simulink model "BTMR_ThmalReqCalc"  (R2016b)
settings: Solver=FixedStepDiscrete  StartTime=0.0  StopTime=10.0  FixedStep=0.1  RelTol=1e-3  EnableMultiTasking=on
undefined symbols (not defined in the file or in its folder): BMS_cntThmStbNum_C, BTMR_cntThmalReqVal_C, BTMR_flgCoolPwrCal_C, BTMR_pChrgClntPwrLv1_C, BTMR_pChrgClntPwrLv2_C, BTMR_pChrgClntPwrLv3_C, BTMR_pChrgClntPwrLv4_C, BTMR_pChrgClntPwrLv5_C, BTMR_pChrgClntPwrLv6_C, BTMR_pCoolPwrVal_C, BTMR_pHtgACPwrReq_C, BTMR_pHtgDCPwrReq_C, BTMR_pHtgDrvPwrReq_C, BTMR_pHtgsStage1_CUR, BTMR_pHtgsStage2_CUR, BTMR_pNormClntPwrLv1_C, BTMR_pNormClntPwrLv2_C, BTMR_pNormClntPwrLv3_C, BTMR_r861BrsDrvSoc_C, BTMR_r861HtgDrvSoc_C, BTMR_r891BrsDrvSoc_C, BTMR_r891HtgDrvSoc_C, BTMR_rCoolClbFlg_C, BTMR_rFlashClbFlg_C, BTMR_rHeatClbFlg_C, BTMR_t861BrsDiffLv0Temp_C, BTMR_t861BrsDiffLv1Temp_C, BTMR_t861CoolChrgAces2Temp_C, BTMR_t861CoolChrgAces3Temp_C, BTMR_t861CoolChrgAcesTemp_C, BTMR_t861CoolChrgDiffDebTemp_C, BTMR_t861CoolChrgEndDiffTemp_C, BTMR_t861CoolChrgExitLv2Temp_C, BTMR_t861CoolChrgExitLv3Temp_C, BTMR_t861CoolChrgExitTemp_C, BTMR_t861CoolChrgIntLv0Temp_C, BTMR_t861CoolChrgIntLv1Temp_C, BTMR_t861CoolChrgIntLv2Temp_C, BTMR_t861CoolChrgIntLv3Temp_C, BTMR_t861CoolChrgIntLv4Temp_C, BTMR_t861CoolChrgIntLv5Temp_C, BTMR_t861CoolDCDebTemp_C, BTMR_t861CoolNormAcesTemp_C, BTMR_t861CoolNormDiffDebTemp_C, BTMR_t861CoolNormEndDiffTemp_C, BTMR_t861CoolNormExitLv2Temp_C, BTMR_t861CoolNormExitLv3Temp_C, BTMR_t861CoolNormExitTemp_C, BTMR_t861CoolNormIntLv0Temp_C, BTMR_t861CoolNormIntLv1Temp_C, BTMR_t861CoolNormLv2Temp_C, BTMR_t861CoolNormLv3Temp_C, BTMR_t861HtgACDiffDebTemp_C, BTMR_t861HtgACEndDiffTemp_C, BTMR_t861HtgACStartHiTemp_C, BTMR_t861HtgACStartLoTemp_C, BTMR_t861HtgACStopTemp_C, BTMR_t861HtgDCDiffDebTemp_C, BTMR_t861HtgDCEndDiffTemp_C, BTMR_t861HtgDCIntLv0Temp_C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
libraries: AIWAYS_Powertrain_BMS_lib x78, simulink x9
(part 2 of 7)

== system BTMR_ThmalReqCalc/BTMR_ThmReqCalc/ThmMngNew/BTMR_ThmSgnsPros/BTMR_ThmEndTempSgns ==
  BSPR_tCellTempMin : Inport
  BSPR_tCellTempMax : Inport  Port=2
  BCMR_bAcChrgHeatFbd : Inport  Port=3
  DSMR_stFaultRank : Inport  Port=4
  BMCR_stBmsModeCtrl : Inport  Port=5
  COMR_bLeadAcidChgHvOn : Inport  Port=6
  BTMR_flgBMSSgns : Inport  Port=7
  BTMR_CoolChrgThmEndCalc : Subsystem
  BTMR_CoolNormThmEndCalc : Subsystem
  BTMR_HtgACThmEndCalc : Subsystem
  BTMR_HtgDCThmEndCalc : Subsystem
  BTMR_HtgDrvThmEndCalc : Subsystem
  BTMR_ThmEndComCalc : Subsystem
  Bus Creator : BusCreator  Inputs=6
  Logical Operator{1..4,10} (5 alike) : Logic  Operator=OR  AllPortsSameDT=off  OutDataTypeStr=boolean
  BTMR_flgThmEndSgns : Outport
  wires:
  BMCR_stBmsModeCtrl/1 -> BTMR_ThmEndComCalc/1(BMCR_stBmsModeCtrl)
  DSMR_stFaultRank/1 -> BTMR_ThmEndComCalc/2(DSMR_stFaultRank)
  BTMR_ThmEndComCalc/1(BTMR_ThmEndCom) -> Logical Operator10/1, Logical Operator4/1, Logical Operator3/1, Logical Operator2/1, Logical Operator1/1, Bus Creator/1  "BTMR_flgBrsThmEnd"
  BTMR_flgBMSSgns/1 -> BTMR_CoolChrgThmEndCalc/1(BTMR_flgBMSSgns), BTMR_CoolNormThmEndCalc/1(BTMR_flgBMSSgns), BTMR_HtgDrvThmEndCalc/1(BTMR_flgBMSSgns), BTMR_HtgACThmEndCalc/1(BTMR_flgBMSSgns), BTMR_HtgDCThmEndCalc/1(BTMR_flgBMSSgns)
  BSPR_tCellTempMax/1 -> BTMR_CoolChrgThmEndCalc/2(BSPR_tCellTempMax), BTMR_CoolNormThmEndCalc/2(BSPR_tCellTempMax), BTMR_HtgDrvThmEndCalc/2(BSPR_tCellTempMax), BTMR_HtgACThmEndCalc/2(BSPR_tCellTempMax), BTMR_HtgDCThmEndCalc/2(BSPR_tCellTempMax)
  BSPR_tCellTempMin/1 -> BTMR_CoolChrgThmEndCalc/3(BSPR_tCellTempMin), BTMR_CoolNormThmEndCalc/3(BSPR_tCellTempMin), BTMR_HtgDrvThmEndCalc/3(BSPR_tCellTempMin), BTMR_HtgACThmEndCalc/3(BSPR_tCellTempMin), BTMR_HtgDCThmEndCalc/3(BSPR_tCellTempMin)
  BTMR_HtgDCThmEndCalc/1(BTMR_HtgDCThmEnd) -> Logical Operator10/2
  BTMR_HtgACThmEndCalc/1(BTMR_HtgACThmEnd) -> Logical Operator1/2
  BTMR_HtgDrvThmEndCalc/1(BTMR_HtgDrvThmEnd) -> Logical Operator2/2
  BTMR_CoolNormThmEndCalc/1(BTMR_CoolNormThmEnd) -> Logical Operator3/2
  BTMR_CoolChrgThmEndCalc/1(BTMR_CoolChrgThmEnd) -> Logical Operator4/2
  Logical Operator10/1 -> Bus Creator/2  "BTMR_flgHtgDCThmEnd"
  Logical Operator1/1 -> Bus Creator/3  "BTMR_flgHtgACThmEnd"
  Logical Operator2/1 -> Bus Creator/4  "BTMR_flgHtgDrvThmEnd"
  Logical Operator3/1 -> Bus Creator/5  "BTMR_flgCoolNormThmEnd"
  Logical Operator4/1 -> Bus Creator/6  "BTMR_flgCoolChrgThmEnd"
  Bus Creator/1 -> BTMR_flgThmEndSgns/1  "BTMR_flgThmEndSgns"
  COMR_bLeadAcidChgHvOn/1 -> BTMR_ThmEndComCalc/3(COMR_bLeadAcidChgHvOn)
  BCMR_bAcChrgHeatFbd/1 -> BTMR_HtgACThmEndCalc/4(BCMR_bAcChrgHeatFbd)

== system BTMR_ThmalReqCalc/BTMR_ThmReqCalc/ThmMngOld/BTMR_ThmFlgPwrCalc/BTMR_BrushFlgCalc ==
  stBrsSts : Inport
  Constant1 : Constant  Value=enmThmBrsFlg.INACTIVE  OutDataTypeStr=Enum: enmThmBrsFlg
  Constant2 : Constant  Value=BTMR_cntThmalReqVal_C
  Constant21 : Constant  Value=enmThmBrsSts.ACTIVE  OutDataTypeStr=Enum: enmThmBrsSts
  Constant3 : Constant  Value=enmThmBrsFlg.ACTIVE  OutDataTypeStr=Enum: enmThmBrsFlg
  Data Type Conversion : DataTypeConversion  OutDataTypeStr=uint8
  Data Type Conversion1 : DataTypeConversion  OutDataTypeStr=uint8
  Data Type Conversion2 : DataTypeConversion  OutDataTypeStr=uint8
  Relational Operator7 : RelationalOperator  Operator===  OutDataTypeStr=boolean  RndMeth=Simplest
  Stable_Calc1 : Subsystem
  Switch1 : Switch  Criteria=u2 ~= 0
  BTMR_flgBrsPwrReq : Outport
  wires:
  Data Type Conversion2/1 -> Switch1/3
  stBrsSts/1 -> Relational Operator7/1
  Data Type Conversion1/1 -> Switch1/1
  Relational Operator7/1 -> Stable_Calc1/1(source_Uint)
  Constant21/1 -> Data Type Conversion/1
  Switch1/1 -> BTMR_flgBrsPwrReq/1
  Data Type Conversion/1 -> Relational Operator7/2
  Constant3/1 -> Data Type Conversion1/1
  Constant1/1 -> Data Type Conversion2/1
  Constant2/1 -> Stable_Calc1/2(cntStable)
  Stable_Calc1/1(stableOut) -> Switch1/2

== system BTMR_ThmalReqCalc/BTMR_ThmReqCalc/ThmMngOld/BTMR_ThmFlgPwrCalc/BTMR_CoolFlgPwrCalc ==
  BTMR_flgBrsPwrReq : Inport
  stCoolSts : Inport  Port=2
  BTMR_flgCoolTempSgns : Inport  Port=3
  BTMR_CoolChrgFlgPwrCalc : Subsystem
  BTMR_CoolNormFlgPwrCalc : Subsystem
  BTMR_flgPow_Out : Subsystem
  Bus Selector1 : BusSelector  OutputSignals=BTMR_flgCoolNormTempSgns,BTMR_flgCoolChrgTempSgns
  Constant1 : Constant  Value=enmThmCoolSts.CoolChrg  OutDataTypeStr=Enum: enmThmCoolSts
  Constant13 : Constant  Value=enmThmCoolSts.CoolNorm  OutDataTypeStr=Enum: enmThmCoolSts
  Data Type Conversion : DataTypeConversion  OutDataTypeStr=uint8
  Data Type Conversion1 : DataTypeConversion  OutDataTypeStr=uint8
  Merge : Merge
  Merge1 : Merge
  Relational Operator2 : RelationalOperator  Operator===  OutDataTypeStr=boolean  RndMeth=Simplest
  Relational Operator3 : RelationalOperator  Operator===  OutDataTypeStr=boolean  RndMeth=Simplest
  BTMR_flgClntPwrReq : Outport
  BTMR_pClntPwrReq : Outport  Port=2
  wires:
  Relational Operator3/1 -> BTMR_CoolChrgFlgPwrCalc/Enable
  stCoolSts/1 -> [stCoolSts], Relational Operator2/1, Relational Operator3/1
  Data Type Conversion1/1 -> Relational Operator3/2
  Relational Operator2/1 -> BTMR_CoolNormFlgPwrCalc/Enable
  Constant13/1 -> Data Type Conversion/1
  BTMR_flgCoolTempSgns/1 -> Bus Selector1/1
  BTMR_flgPow_Out/1(BTMR_flgClntPwrReq) -> BTMR_flgClntPwrReq/1
  BTMR_flgPow_Out/2(BTMR_pClntPwrReq) -> BTMR_pClntPwrReq/1
  Bus Selector1/1 -> BTMR_CoolNormFlgPwrCalc/1(BTMR_flgCoolNormTempSgns)  "<BTMR_flgCoolNormTempSgns>"
  Bus Selector1/2 -> BTMR_CoolChrgFlgPwrCalc/1(BTMR_flgCoolChrgTempSgns)  "<BTMR_flgCoolChrgTempSgns>"
  BTMR_flgBrsPwrReq/1 -> BTMR_flgPow_Out/2(BTMR_flgBrsPwrReq)
  Data Type Conversion/1 -> Relational Operator2/2
  Constant1/1 -> Data Type Conversion1/1
  BTMR_CoolNormFlgPwrCalc/1(BTMR_flgClntPwrReq) -> Merge/1
  BTMR_CoolChrgFlgPwrCalc/1(BTMR_flgClntPwrReq) -> Merge/2
  BTMR_CoolNormFlgPwrCalc/2(BTMR_pClntPwrReq) -> Merge1/1
  Merge/1 -> BTMR_flgPow_Out/3(BTMR_flgClntPwrReqMerge)
  BTMR_CoolChrgFlgPwrCalc/2(BTMR_pClntPwrReq) -> Merge1/2
  [stCoolSts] -> BTMR_flgPow_Out/1(stCoolSts)
  Merge1/1 -> BTMR_flgPow_Out/4(BTMR_pClntPwrReqMerge)

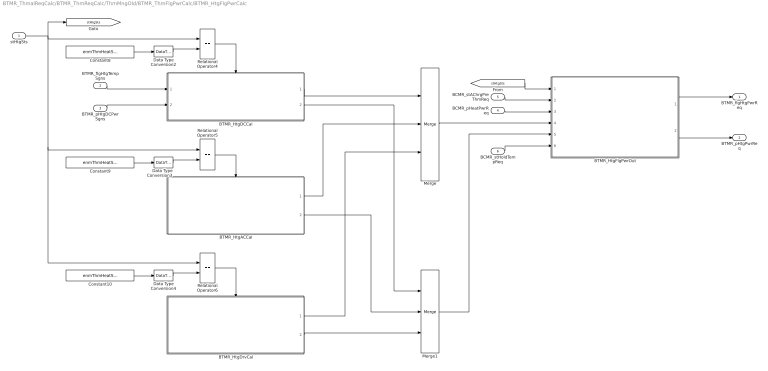
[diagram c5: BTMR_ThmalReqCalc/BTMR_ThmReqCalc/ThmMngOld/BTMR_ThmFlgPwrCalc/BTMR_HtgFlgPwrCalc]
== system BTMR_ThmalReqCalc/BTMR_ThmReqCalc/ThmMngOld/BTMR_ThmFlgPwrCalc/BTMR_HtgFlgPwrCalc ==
  stHtgSts : Inport
  BTMR_flgHtgTempSgns : Inport  Port=2
  BTMR_pHtgDCPwrSgns : Inport  Port=3
  BCMR_pHeatPwrReq : Inport  Port=4
  BCMR_stAChrgPreThmReq : Inport  Port=5
  BCMR_stHoldTempReq : Inport  Port=6
  BTMR_HtgACCal : Subsystem
  BTMR_HtgDCCal : Subsystem
  BTMR_HtgDrvCal : Subsystem
  BTMR_HtgFlgPwrOut : Subsystem
  Constant10 : Constant  Value=enmThmHeatSts.HeatDrv  OutDataTypeStr=Enum: enmThmHeatSts
  Constant8 : Constant  Value=enmThmHeatSts.HeatDC  OutDataTypeStr=Enum: enmThmHeatSts
  Constant9 : Constant  Value=enmThmHeatSts.HeatAC  OutDataTypeStr=Enum: enmThmHeatSts
  Data Type Conversion2 : DataTypeConversion  OutDataTypeStr=uint8
  Data Type Conversion3 : DataTypeConversion  OutDataTypeStr=uint8
  Data Type Conversion4 : DataTypeConversion  OutDataTypeStr=uint8
  Merge : Merge  Inputs=3
  Merge1 : Merge  Inputs=3
  Relational Operator4 : RelationalOperator  Operator===  OutDataTypeStr=boolean  RndMeth=Simplest
  Relational Operator5 : RelationalOperator  Operator===  OutDataTypeStr=boolean  RndMeth=Simplest
  Relational Operator6 : RelationalOperator  Operator===  OutDataTypeStr=boolean  RndMeth=Simplest
  BTMR_flgHtgPwrReq : Outport
  BTMR_pHtgPwrReq : Outport  Port=2
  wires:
  stHtgSts/1 -> [stHtgSts], Relational Operator6/1, Relational Operator5/1, Relational Operator4/1
  Relational Operator6/1 -> BTMR_HtgDrvCal/Enable
  BTMR_flgHtgTempSgns/1 -> BTMR_HtgDCCal/1(BTMR_flgHtgDCCalSgns)
  BTMR_pHtgDCPwrSgns/1 -> BTMR_HtgDCCal/2(BTMR_pHtgDCPowCur)
  Relational Operator4/1 -> BTMR_HtgDCCal/Enable
  Data Type Conversion2/1 -> Relational Operator4/2
  Constant8/1 -> Data Type Conversion2/1
  Data Type Conversion3/1 -> Relational Operator5/2
  Constant9/1 -> Data Type Conversion3/1
  Data Type Conversion4/1 -> Relational Operator6/2
  Constant10/1 -> Data Type Conversion4/1
  Relational Operator5/1 -> BTMR_HtgACCal/Enable
  BTMR_HtgDCCal/1(BTMR_flgHtgPwrReq) -> Merge/1
  BTMR_HtgACCal/1(BTMR_flgHtgPwrReq) -> Merge/2
  BTMR_HtgDrvCal/1(BTMR_flgHtgPwrReq) -> Merge/3
  BTMR_HtgDrvCal/2(BTMR_pHtgPwrReq) -> Merge1/3
  BTMR_HtgDCCal/2(BTMR_pHtgPwrReq) -> Merge1/1
  BTMR_HtgACCal/2(BTMR_pHtgPwrReq) -> Merge1/2
  BCMR_stAChrgPreThmReq/1 -> BTMR_HtgFlgPwrOut/2(BCMR_stAChrgPreThmReq)
  Merge/1 -> BTMR_HtgFlgPwrOut/4(BTMR_flgHtgPwrReqMerge)
  [stHtgSts] -> BTMR_HtgFlgPwrOut/1(stHtgSts)
  BCMR_pHeatPwrReq/1 -> BTMR_HtgFlgPwrOut/3(BCMR_pHeatPwrReq)
  Merge1/1 -> BTMR_HtgFlgPwrOut/5(BTMR_pHtgPwrReqMerge)
  BTMR_HtgFlgPwrOut/1(BTMR_flgHtgPwrReq) -> BTMR_flgHtgPwrReq/1
  BTMR_HtgFlgPwrOut/2(BTMR_pHtgPwrReq) -> BTMR_pHtgPwrReq/1
  BCMR_stHoldTempReq/1 -> BTMR_HtgFlgPwrOut/6(BCMR_stHoldTempReq)

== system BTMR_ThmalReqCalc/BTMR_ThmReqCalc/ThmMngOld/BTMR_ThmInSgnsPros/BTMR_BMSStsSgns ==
  COMR_bLeadAcidChgHvOn : Inport
  BMCR_stBmsModeCtrl : Inport  Port=2
  BSER_rSoc : Inport  Port=3
  BTMR_BmsStsCalc : Subsystem
  BTMR_SOCStsCalc : Subsystem
  BTMR_flgBMSSgns : Outport
  BTMR_flgSOCSgns : Outport  Port=2
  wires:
  BSER_rSoc/1 -> BTMR_SOCStsCalc/1(BSER_rSoc)
  BMCR_stBmsModeCtrl/1 -> BTMR_BmsStsCalc/1(BMCR_stBmsModeCtrl)
  BTMR_SOCStsCalc/1(BTMR_flgSOCSgns) -> BTMR_flgSOCSgns/1
  BTMR_BmsStsCalc/1(BTMR_flgBMSSgns) -> BTMR_flgBMSSgns/1
  COMR_bLeadAcidChgHvOn/1 -> BTMR_BmsStsCalc/2(COMR_bLeadAcidChgHvOn)

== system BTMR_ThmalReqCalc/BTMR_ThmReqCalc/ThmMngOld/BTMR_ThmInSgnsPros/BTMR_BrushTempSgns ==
  BSPR_tCellTempMin : Inport
  BSPR_tCellTempMax : Inport  Port=2
  BSPR_tClntUsT : Inport  Port=3
  BTMR_BrsDnaTempCalc : Subsystem
  BTMR_BrsEna1TempCalc : Subsystem
  BTMR_BrsEna2TempCalc : Subsystem
  BTMR_BrsEna3TempCalc : Subsystem
  BTMR_BrsIntEna1TempCalc : Subsystem
  BTMR_BrsIntEna2TempCalc : Subsystem
  BTMR_BrsIntEna3TempCalc : Subsystem
  BTMR_BrsStartTempCalc : Subsystem
  Bus Creator : BusCreator  Inputs=2
  Bus Creator1 : BusCreator  Inputs=3
  Bus Creator2 : BusCreator  Inputs=3
  Bus Creator3 : BusCreator  Inputs=3
  BTMR_flgBrsTempSgns : Outport
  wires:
  BTMR_BrsEna2TempCalc/1(BTMR_flgBrsEna2Temp) -> Bus Creator1/2  "BTMR_flgBrsEna2Temp"
  BTMR_BrsEna1TempCalc/1(BTMR_flgBrsEna1Temp) -> Bus Creator1/1  "BTMR_flgBrsEna1Temp"
  BTMR_BrsStartTempCalc/1(BTMR_flgBrsStartTemp) -> Bus Creator/1  "BTMR_flgBrsStartTemp"
  BSPR_tCellTempMin/1 -> BTMR_BrsEna3TempCalc/1(BSPR_tCellTempMin), BTMR_BrsEna2TempCalc/1(BSPR_tCellTempMin), BTMR_BrsEna1TempCalc/1(BSPR_tCellTempMin), BTMR_BrsDnaTempCalc/1(BSPR_tCellTempMin), BTMR_BrsStartTempCalc/1(BSPR_tCellTempMin)
  BSPR_tCellTempMax/1 -> BTMR_BrsEna3TempCalc/2(BSPR_tCellTempMax), BTMR_BrsEna2TempCalc/2(BSPR_tCellTempMax), BTMR_BrsEna1TempCalc/2(BSPR_tCellTempMax), BTMR_BrsDnaTempCalc/2(BSPR_tCellTempMax), BTMR_BrsStartTempCalc/2(BSPR_tCellTempMax)
  BSPR_tClntUsT/1 -> BTMR_BrsIntEna3TempCalc/1(BSPR_tClntUsT), BTMR_BrsStartTempCalc/3(BSPR_tClntUsT), BTMR_BrsIntEna1TempCalc/1(BSPR_tClntUsT), BTMR_BrsIntEna2TempCalc/1(BSPR_tClntUsT)
  BTMR_BrsDnaTempCalc/1(BTMR_flgBrsDnaTemp) -> Bus Creator/2  "BTMR_flgBrsDnaTemp"
  BTMR_BrsEna3TempCalc/1(BTMR_flgBrsEna3Temp) -> Bus Creator1/3  "BTMR_flgBrsEna3Temp"
  BTMR_BrsIntEna1TempCalc/1(BTMR_flgBrsIntEna1Temp) -> Bus Creator2/1  "BTMR_flgBrsIntEna1Temp"
  BTMR_BrsIntEna2TempCalc/1(BTMR_flgBrsIntEna2Temp) -> Bus Creator2/2  "BTMR_flgBrsIntEna2Temp"
  BTMR_BrsIntEna3TempCalc/1(BTMR_flgBrsIntEna3Temp) -> Bus Creator2/3  "BTMR_flgBrsIntEna3Temp"
  Bus Creator/1 -> Bus Creator3/1  "BTMR_flgBrsInTempSgns"
  Bus Creator1/1 -> Bus Creator3/2  "BTMR_flgBrsEnTempSgns"
  Bus Creator2/1 -> Bus Creator3/3  "BTMR_flgBrsIntTempSgns"
  Bus Creator3/1 -> BTMR_flgBrsTempSgns/1

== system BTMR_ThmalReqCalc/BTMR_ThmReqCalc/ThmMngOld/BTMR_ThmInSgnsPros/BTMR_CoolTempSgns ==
  BSPR_tCellTempMax : Inport
  BSPR_tClntUsT : Inport  Port=2
  BTMR_CoolChrgTempCalc : Subsystem
  BTMR_CoolNormTempCalc : Subsystem
  Bus Creator : BusCreator  Inputs=2
  BTMR_flgCoolTempSgns : Outport
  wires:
  BSPR_tCellTempMax/1 -> BTMR_CoolChrgTempCalc/1(BSPR_tCellTempMax), BTMR_CoolNormTempCalc/1(BSPR_tCellTempMax)
  BSPR_tClntUsT/1 -> BTMR_CoolChrgTempCalc/2(BSPR_tClntUsT), BTMR_CoolNormTempCalc/2(BSPR_tClntUsT)
  Bus Creator/1 -> BTMR_flgCoolTempSgns/1  "BTMR_flgCoolTempSgns"
  BTMR_CoolChrgTempCalc/1(BTMR_flgCoolChrgTempSgns) -> Bus Creator/2
  BTMR_CoolNormTempCalc/1(BTMR_flgCoolNormTempSgns) -> Bus Creator/1

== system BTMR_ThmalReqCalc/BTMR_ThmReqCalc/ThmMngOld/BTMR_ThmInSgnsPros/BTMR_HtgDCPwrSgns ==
  COMR_tEnvT : Inport
  2-D Lookup Table : Lookup_n-D  NumberOfTableDimensions=1  BreakpointsForDimension1=BTMR_tEnvTStage1_A  BreakpointsForDimension2=[1:3]  Table=BTMR_pHtgsStage1_CUR  ExtrapMethod=Clip  UseLastTableValue=on  InternalRulePriority=Speed  RndMeth=Simplest
  2-D Lookup Table1 : Lookup_n-D  NumberOfTableDimensions=1  BreakpointsForDimension1=BTMR_tEnvTStage2_A  BreakpointsForDimension2=[1:3]  Table=BTMR_pHtgsStage2_CUR  ExtrapMethod=Clip  UseLastTableValue=on  InternalRulePriority=Speed  RndMeth=Simplest
  Bus Creator1 : BusCreator  Inputs=2
  BTMR_pHtgDCPwrSgns : Outport
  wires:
  COMR_tEnvT/1 -> 2-D Lookup Table1/1, 2-D Lookup Table/1
  2-D Lookup Table/1 -> Bus Creator1/1  "BTMR_pHtgDCPowCur1"
  2-D Lookup Table1/1 -> Bus Creator1/2  "BTMR_pHtgDCPowCur2"
  Bus Creator1/1 -> BTMR_pHtgDCPwrSgns/1

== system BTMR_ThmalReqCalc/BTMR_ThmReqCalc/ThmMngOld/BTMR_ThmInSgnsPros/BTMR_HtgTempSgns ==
  BSPR_tCellTempMin : Inport
  BSPR_tCellTempMax : Inport  Port=2
  BSPR_tClntUsT : Inport  Port=3
  BTMR_HtgACTempCalc : Subsystem
  BTMR_HtgDCTempCalc : Subsystem
  BTMR_HtgDrvTempCalc : Subsystem
  Bus Creator : BusCreator  Inputs=3
  BTMR_flgHtgTempSgns : Outport
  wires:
  BSPR_tCellTempMin/1 -> BTMR_HtgDrvTempCalc/1(BSPR_tCellTempMin), BTMR_HtgACTempCalc/1(BSPR_tCellTempMin), BTMR_HtgDCTempCalc/1(BSPR_tCellTempMin)
  BSPR_tCellTempMax/1 -> BTMR_HtgDCTempCalc/2(BSPR_tCellTempMax)
  BSPR_tClntUsT/1 -> BTMR_HtgDCTempCalc/3(BSPR_tClntUsT)
  BTMR_HtgACTempCalc/1(BTMR_flgHtgACTempSgns) -> Bus Creator/2
  BTMR_HtgDCTempCalc/1(BTMR_flgHtgDCTempSgns) -> Bus Creator/1
  BTMR_HtgDrvTempCalc/1(BTMR_flgHtgDrvTempSgns) -> Bus Creator/3
  Bus Creator/1 -> BTMR_flgHtgTempSgns/1  "BTMR_flgHtgTempSgns"

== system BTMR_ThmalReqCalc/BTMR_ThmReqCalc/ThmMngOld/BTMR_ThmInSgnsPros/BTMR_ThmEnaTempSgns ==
  BSPR_tCellTempMin : Inport
  BSPR_tCellTempMax : Inport  Port=2
  BTMR_CoolChrgEnaTempCalc : Subsystem
  BTMR_CoolNormEnaTempCalc : Subsystem
  BTMR_HtgACEnaTempCalc : Subsystem
  BTMR_HtgDCEnaTempCalc : Subsystem
  BTMR_HtgDrvEnaTempCalc : Subsystem
  Bus Creator : BusCreator  Inputs=5
  Bus Creator1 : BusCreator  Inputs=2
  Bus Selector{,1..4} (5 alike) : BusSelector  OutputSignals=BSPR_tCellTempMin,BSPR_tCellTempMax
  BTMR_flgThmEnaTempSgns : Outport
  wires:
  Bus Creator/1 -> BTMR_flgThmEnaTempSgns/1
  Bus Selector3/2 -> BTMR_CoolChrgEnaTempCalc/2(BSPR_tCellTempMax)  "<BSPR_tCellTempMax>"
  BTMR_CoolChrgEnaTempCalc/1(BTMR_flgCoolChrgEnaTemp) -> Bus Creator/4  "BTMR_CoolChrgEnaTemp"
  BTMR_CoolNormEnaTempCalc/1(BTMR_flgCoolNormEnaTemp) -> Bus Creator/5  "BTMR_CoolNormEnaTemp"
  BTMR_HtgDrvEnaTempCalc/1(BTMR_flgHtgDrvEnaTemp) -> Bus Creator/3  "BTMR_HtgDrvEnaTemp"
  BTMR_HtgDCEnaTempCalc/1(BTMR_flgHtgDCEnaTemp) -> Bus Creator/1  "BTMR_HtgDCEnaTemp"
  BTMR_HtgACEnaTempCalc/1(BTMR_flgHtgACEnaTemp) -> Bus Creator/2  "BTMR_HtgACEnaTemp"
  BSPR_tCellTempMin/1 -> Bus Creator1/1
  BSPR_tCellTempMax/1 -> Bus Creator1/2
  Bus Creator1/1 -> Bus Selector4/1, Bus Selector3/1, Bus Selector2/1, Bus Selector1/1, Bus Selector/1
  Bus Selector1/1 -> BTMR_HtgDCEnaTempCalc/1(BSPR_tCellTempMin)  "<BSPR_tCellTempMin>"
  Bus Selector/1 -> BTMR_HtgACEnaTempCalc/1(BSPR_tCellTempMin)  "<BSPR_tCellTempMin>"
  Bus Selector2/1 -> BTMR_HtgDrvEnaTempCalc/1(BSPR_tCellTempMin)  "<BSPR_tCellTempMin>"
  Bus Selector1/2 -> BTMR_HtgDCEnaTempCalc/2(BSPR_tCellTempMax)  "<BSPR_tCellTempMax>"
  Bus Selector/2 -> BTMR_HtgACEnaTempCalc/2(BSPR_tCellTempMax)  "<BSPR_tCellTempMax>"
  Bus Selector2/2 -> BTMR_HtgDrvEnaTempCalc/2(BSPR_tCellTempMax)  "<BSPR_tCellTempMax>"
  Bus Selector3/1 -> BTMR_CoolChrgEnaTempCalc/1(BSPR_tCellTempMin)  "<BSPR_tCellTempMin>"
  Bus Selector4/2 -> BTMR_CoolNormEnaTempCalc/2(BSPR_tCellTempMax)  "<BSPR_tCellTempMax>"
  Bus Selector4/1 -> BTMR_CoolNormEnaTempCalc/1(BSPR_tCellTempMin)  "<BSPR_tCellTempMin>"

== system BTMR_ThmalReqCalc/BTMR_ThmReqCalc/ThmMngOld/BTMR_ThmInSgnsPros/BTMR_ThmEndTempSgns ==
  BSPR_tCellTempMin : Inport
  BSPR_tCellTempMax : Inport  Port=2
  BCMR_bAcChrgHeatFbd : Inport  Port=3
  DSMR_stFaultRank : Inport  Port=4
  BMCR_stBmsModeCtrl : Inport  Port=5
  COMR_bLeadAcidChgHvOn : Inport  Port=6
  BTMR_flgBMSSgns : Inport  Port=7
  BTMR_CoolChrgThmEndCalc : Subsystem
  BTMR_CoolNormThmEndCalc : Subsystem
  BTMR_HtgACThmEndCalc : Subsystem
  BTMR_HtgDCThmEndCalc : Subsystem
  BTMR_HtgDrvThmEndCalc : Subsystem
  BTMR_ThmEndComCalc : Subsystem
  Bus Creator : BusCreator  Inputs=6
  Logical Operator{1..4,10} (5 alike) : Logic  Operator=OR  AllPortsSameDT=off  OutDataTypeStr=boolean
  BTMR_flgThmEndSgns : Outport
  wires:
  BMCR_stBmsModeCtrl/1 -> BTMR_ThmEndComCalc/1(BMCR_stBmsModeCtrl)
  DSMR_stFaultRank/1 -> BTMR_ThmEndComCalc/2(DSMR_stFaultRank)
  BTMR_ThmEndComCalc/1(BTMR_ThmEndCom) -> Logical Operator10/1, Logical Operator4/1, Logical Operator3/1, Logical Operator2/1, Logical Operator1/1, Bus Creator/1  "BTMR_flgBrsThmEnd"
  BTMR_flgBMSSgns/1 -> BTMR_CoolChrgThmEndCalc/1(BTMR_flgBMSSgns), BTMR_CoolNormThmEndCalc/1(BTMR_flgBMSSgns), BTMR_HtgDrvThmEndCalc/1(BTMR_flgBMSSgns), BTMR_HtgACThmEndCalc/1(BTMR_flgBMSSgns), BTMR_HtgDCThmEndCalc/1(BTMR_flgBMSSgns)
  BSPR_tCellTempMax/1 -> BTMR_CoolChrgThmEndCalc/2(BSPR_tCellTempMax), BTMR_CoolNormThmEndCalc/2(BSPR_tCellTempMax), BTMR_HtgDrvThmEndCalc/2(BSPR_tCellTempMax), BTMR_HtgACThmEndCalc/2(BSPR_tCellTempMax), BTMR_HtgDCThmEndCalc/2(BSPR_tCellTempMax)
  BSPR_tCellTempMin/1 -> BTMR_CoolChrgThmEndCalc/3(BSPR_tCellTempMin), BTMR_CoolNormThmEndCalc/3(BSPR_tCellTempMin), BTMR_HtgDrvThmEndCalc/3(BSPR_tCellTempMin), BTMR_HtgACThmEndCalc/3(BSPR_tCellTempMin), BTMR_HtgDCThmEndCalc/3(BSPR_tCellTempMin)
  BTMR_HtgDCThmEndCalc/1(BTMR_HtgDCThmEnd) -> Logical Operator10/2
  BTMR_HtgACThmEndCalc/1(BTMR_HtgACThmEnd) -> Logical Operator1/2
  BTMR_HtgDrvThmEndCalc/1(BTMR_HtgDrvThmEnd) -> Logical Operator2/2
  BTMR_CoolNormThmEndCalc/1(BTMR_CoolNormThmEnd) -> Logical Operator3/2
  BTMR_CoolChrgThmEndCalc/1(BTMR_CoolChrgThmEnd) -> Logical Operator4/2
  Logical Operator10/1 -> Bus Creator/2  "BTMR_flgHtgDCThmEnd"
  Logical Operator1/1 -> Bus Creator/3  "BTMR_flgHtgACThmEnd"
  Logical Operator2/1 -> Bus Creator/4  "BTMR_flgHtgDrvThmEnd"
  Logical Operator3/1 -> Bus Creator/5  "BTMR_flgCoolNormThmEnd"
  Logical Operator4/1 -> Bus Creator/6  "BTMR_flgCoolChrgThmEnd"
  Bus Creator/1 -> BTMR_flgThmEndSgns/1  "BTMR_flgThmEndSgns"
  COMR_bLeadAcidChgHvOn/1 -> BTMR_ThmEndComCalc/3(COMR_bLeadAcidChgHvOn)
  BCMR_bAcChrgHeatFbd/1 -> BTMR_HtgACThmEndCalc/4(BCMR_bAcChrgHeatFbd)

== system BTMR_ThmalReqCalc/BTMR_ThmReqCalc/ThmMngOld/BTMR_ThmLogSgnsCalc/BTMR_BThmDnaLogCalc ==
  BTMR_flgSOCSgns : Inport
  BTMR_flgBrsTempSgns : Inport  Port=2
  BTMR_flgHtgTempSgns : Inport  Port=3
  BTMR_flgCoolTempSgns : Inport  Port=4
  BTMR_BrsDnaCalc : Subsystem
  BTMR_CoolDnaCalc : Subsystem
  BTMR_HtgDnaCalc : Subsystem
  Bus Creator : BusCreator  Inputs=6
  BTMR_flgBThmDnaSgns : Outport
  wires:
  BTMR_CoolDnaCalc/2(BTMR_flgCoolChrgDna) -> Bus Creator/6  "BTMR_flgCoolChrgDna"
  BTMR_CoolDnaCalc/1(BTMR_flgCoolNormDna) -> Bus Creator/5  "BTMR_flgCoolNormDna"
  BTMR_HtgDnaCalc/3(BTMR_flgHtgDrvDna) -> Bus Creator/4  "BTMR_flgHtgDrvDna"
  BTMR_HtgDnaCalc/2(BTMR_flgHtgACDna) -> Bus Creator/3  "BTMR_flgHtgACDna"
  BTMR_HtgDnaCalc/1(BTMR_flgHtgDCDna) -> Bus Creator/2  "BTMR_flgHtgDCDna"
  BTMR_flgCoolTempSgns/1 -> BTMR_CoolDnaCalc/1(BTMR_flgCoolLogSgns)
  BTMR_flgHtgTempSgns/1 -> BTMR_HtgDnaCalc/1(BTMR_flgHtgLogSgns)
  BTMR_BrsDnaCalc/1(BTMR_flgBrsDna) -> Bus Creator/1  "BTMR_flgBrsDna"
  Bus Creator/1 -> BTMR_flgBThmDnaSgns/1  "BTMR_flgBThmDnaSgns"
  BTMR_flgBrsTempSgns/1 -> BTMR_BrsDnaCalc/1(BTMR_flgBrsLogSgns)
  BTMR_flgSOCSgns/1 -> BTMR_HtgDnaCalc/2(BTMR_flgSOCSgns)

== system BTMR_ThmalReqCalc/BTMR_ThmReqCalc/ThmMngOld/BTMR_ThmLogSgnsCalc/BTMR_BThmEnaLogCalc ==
  BTMR_flgBrsLogSgns : Inport
  BTMR_flgHtgLogSgns : Inport  Port=2
  BTMR_flgCoolLogSgns : Inport  Port=3
  BTMR_flgSOCSgns : Inport  Port=4
  BTMR_BrsEnaCalc : Subsystem
  BTMR_CoolEnaCalc : Subsystem
  BTMR_HtgEnaCalc : Subsystem
  Bus Creator : BusCreator  Inputs=6
  BTMR_flgBTMREnaSgns : Outport
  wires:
  BTMR_flgBrsLogSgns/1 -> BTMR_BrsEnaCalc/1(BTMR_flgBrsLogSgns)
  Bus Creator/1 -> BTMR_flgBTMREnaSgns/1  "BTMR_flgBTMREnaSgns"
  BTMR_BrsEnaCalc/1(BTMR_flgBrsEna) -> Bus Creator/1
  BTMR_flgHtgLogSgns/1 -> BTMR_HtgEnaCalc/1(BTMR_flgHtgLogSgns)
  BTMR_flgCoolLogSgns/1 -> BTMR_CoolEnaCalc/1(BTMR_flgCoolLogSgns)
  BTMR_HtgEnaCalc/1(BTMR_flgHtgDCEna) -> Bus Creator/2
  BTMR_HtgEnaCalc/2(BTMR_flgHtgACEna) -> Bus Creator/3
  BTMR_HtgEnaCalc/3(BTMR_flgHtgDrvEna) -> Bus Creator/4
  BTMR_CoolEnaCalc/1(BTMR_flgCoolNormEna) -> Bus Creator/5
  BTMR_CoolEnaCalc/2(BTMR_flgCoolChrgEna) -> Bus Creator/6
  BTMR_flgSOCSgns/1 -> BTMR_HtgEnaCalc/2(BTMR_flgSOCSgns)

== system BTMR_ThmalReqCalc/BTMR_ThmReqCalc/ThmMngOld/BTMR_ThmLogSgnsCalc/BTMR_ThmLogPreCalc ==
  BTMR_flgBMSStsSgns : Inport
  BTMR_flgSOCSgns : Inport  Port=2
  BTMR_flgThmEnaTempSgns : Inport  Port=3
  BTMR_flgBrsTempSgns : Inport  Port=4
  BTMR_BrsLogCalc : Subsystem
  BTMR_CoolLogCalc : Subsystem
  BTMR_HtgLogCalc : Subsystem
  BTMR_flgBrsLogSgns : Outport
  BTMR_flgHtgLogSgns : Outport  Port=2
  BTMR_flgCoolLogSgns : Outport  Port=3
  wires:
  BTMR_flgBMSStsSgns/1 -> BTMR_BrsLogCalc/1(BTMR_flgBMSStsSgns)
  BTMR_flgBrsTempSgns/1 -> BTMR_BrsLogCalc/3(BTMR_flgBrsTempSgns)
  BTMR_flgSOCSgns/1 -> BTMR_BrsLogCalc/2(BTMR_flgSOCSgns)
  BTMR_BrsLogCalc/1(BTMR_flgBrsLogSgns) -> BTMR_flgBrsLogSgns/1, BTMR_HtgLogCalc/1(BTMR_flgBrsLogSgns)
  BTMR_CoolLogCalc/1(BTMR_flgCoolLogSgns) -> BTMR_flgCoolLogSgns/1
  BTMR_HtgLogCalc/1(BTMR_flgHtgLogSgns) -> BTMR_flgHtgLogSgns/1, BTMR_CoolLogCalc/1(BTMR_flgHtgLogSgns)
  BTMR_flgThmEnaTempSgns/1 -> BTMR_CoolLogCalc/2(BTMR_flgThmEnaTempSgns), BTMR_HtgLogCalc/2(BTMR_flgThmEnaTempSgns)

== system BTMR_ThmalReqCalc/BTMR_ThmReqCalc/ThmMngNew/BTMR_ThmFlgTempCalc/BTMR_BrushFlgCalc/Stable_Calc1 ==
  source_Uint : Inport
  cntStable : Inport  Port=2
  Chart : Stateflow chart  TreatAsAtomicUnit=on
  Delay1 : Delay  DelayLength=1  InitialCondition=0
  Detect Change : simulink/Logic and Bit Operations/Detect Change  vinit=0  OutDataTypeStr=boolean
  Switch : Switch  Criteria=u2 ~= 0
  stableOut : Outport
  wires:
  source_Uint/1 -> Detect Change/1, Switch/3
  Switch/1 -> stableOut/1, Delay1/1
  Delay1/1 -> Switch/1
  Chart/1(flg_out) -> Switch/2
  cntStable/1 -> Chart/2(cntStable)
  Detect Change/1 -> Chart/1(trigger_in)

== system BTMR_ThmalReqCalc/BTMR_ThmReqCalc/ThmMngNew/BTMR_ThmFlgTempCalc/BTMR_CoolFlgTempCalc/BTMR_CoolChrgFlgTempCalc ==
  BTMR_flgCoolChrgTempSgns : Inport
  Enable : EnablePort  StatesWhenEnabling=reset
  BTMR_ClntTempReqCalc : Subsystem
  BTMR_ClntTempReqFlgCalc : Subsystem
  Bus Selector : BusSelector  OutputSignals=BTMR_flgCoolChrgStage2EnaTemp,BTMR_flgCoolChrgStage3EnaTemp,BTMR_flgCoolChrgStage2ExtTemp,BTMR_flgCoolChrgStage3ExtTemp
  Chart : Stateflow chart  TreatAsAtomicUnit=on
  Constant12 : Constant  Value=BMS_cntThmStbNum_C
  Data Type Conversion : DataTypeConversion  OutDataTypeStr=uint8
  Stable_Calc : Subsystem
  BTMR_flgClntTempReq : Outport  InitialOutput=0
  BTMR_tClntTempReq : Outport  Port=2  InitialOutput=0
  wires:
  BTMR_flgCoolChrgTempSgns/1 -> Bus Selector/1
  Bus Selector/1 -> Chart/1(CoolChrgStage2Ena)  "<BTMR_flgCoolChrgStage2EnaTemp>"
  Bus Selector/2 -> Chart/2(CoolChrgStage3Ena)  "<BTMR_flgCoolChrgStage3EnaTemp>"
  Bus Selector/3 -> Chart/3(CoolChrgStage2Ext)  "<BTMR_flgCoolChrgStage2ExtTemp>"
  Bus Selector/4 -> Chart/4(CoolChrgStage3Ext)  "<BTMR_flgCoolChrgStage3ExtTemp>"
  Chart/1(BTMR_stsClntStg) -> Data Type Conversion/1
  Stable_Calc/1(stableOut) -> BTMR_ClntTempReqCalc/1(BTMR_stsClntStg), BTMR_ClntTempReqFlgCalc/1(BTMR_stsClntStg)
  BTMR_ClntTempReqFlgCalc/1(BTMR_flgClntTempReq) -> BTMR_flgClntTempReq/1
  BTMR_ClntTempReqCalc/1(BTMR_tClntTempReq) -> BTMR_tClntTempReq/1
  Constant12/1 -> Stable_Calc/2(cntStable)
  Data Type Conversion/1 -> Stable_Calc/1(source_Uint)

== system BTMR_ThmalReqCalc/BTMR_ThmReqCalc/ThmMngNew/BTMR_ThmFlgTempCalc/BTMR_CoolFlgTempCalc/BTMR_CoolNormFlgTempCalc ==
  BTMR_flgCoolNormTempSgns : Inport
  Enable : EnablePort  StatesWhenEnabling=reset
  BSER_ClntTempReqCalc : Subsystem
  BSER_ClntTempReqFlgCalc : Subsystem
  Bus Selector : BusSelector  OutputSignals=BTMR_flgCoolNormStage2EnaTemp,BTMR_flgCoolNormStage3EnaTemp,BTMR_flgCoolNormStage2ExtTemp,BTMR_flgCoolNormStage3ExtTemp
  Chart : Stateflow chart  TreatAsAtomicUnit=on
  Constant12 : Constant  Value=BMS_cntThmStbNum_C
  Data Type Conversion : DataTypeConversion  OutDataTypeStr=uint8
  Stable_Calc : Subsystem
  BTMR_flgClntTempReq : Outport  InitialOutput=0
  BTMR_tClntTempReq : Outport  Port=2  InitialOutput=0
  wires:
  BTMR_flgCoolNormTempSgns/1 -> Bus Selector/1
  Bus Selector/1 -> Chart/1(CoolNormStage2Ena)  "<BTMR_flgCoolNormStage2EnaTemp>"
  Bus Selector/2 -> Chart/2(CoolNormStage3Ena)  "<BTMR_flgCoolNormStage3EnaTemp>"
  Bus Selector/3 -> Chart/3(CoolNormStage2Ext)  "<BTMR_flgCoolNormStage2ExtTemp>"
  Bus Selector/4 -> Chart/4(CoolNormStage3Ext)  "<BTMR_flgCoolNormStage3ExtTemp>"
  Chart/1(BTMR_stsClntStg) -> Data Type Conversion/1
  Stable_Calc/1(stableOut) -> BSER_ClntTempReqCalc/1(BTMR_stsClntStg), BSER_ClntTempReqFlgCalc/1(BTMR_stsClntStg)
  BSER_ClntTempReqFlgCalc/1(BTMR_flgClntTempReq) -> BTMR_flgClntTempReq/1
  BSER_ClntTempReqCalc/1(BTMR_tClntTempReq) -> BTMR_tClntTempReq/1
  Constant12/1 -> Stable_Calc/2(cntStable)
  Data Type Conversion/1 -> Stable_Calc/1(source_Uint)

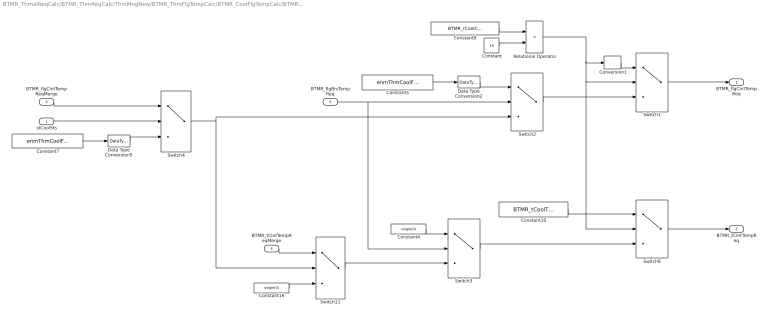
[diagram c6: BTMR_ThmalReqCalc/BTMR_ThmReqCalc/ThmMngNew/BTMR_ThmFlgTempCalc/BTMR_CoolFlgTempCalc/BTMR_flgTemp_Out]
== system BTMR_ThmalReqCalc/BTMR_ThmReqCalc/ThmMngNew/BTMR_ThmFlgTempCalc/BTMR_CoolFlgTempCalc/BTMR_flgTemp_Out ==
  stCoolSts : Inport
  BTMR_flgBrsTempReq : Inport  Port=2
  BTMR_flgClntTempReqMerge : Inport  Port=3
  BTMR_tClntTempReqMerge : Inport  Port=4
  Constant : Constant  Value=10  OutDataTypeStr=single
  Constant10 : Constant  Value=BTMR_tCoolTempClbQnt_C
  Constant16 : Constant  Value=single(0)
  Constant4 : Constant  Value=single(0)
  Constant5 : Constant  Value=enmThmCoolFlg.FLASH  OutDataTypeStr=Enum: enmThmCoolFlg
  Constant7 : Constant  Value=enmThmCoolFlg.INACTIVE  OutDataTypeStr=Enum: enmThmCoolFlg
  Constant9 : Constant  Value=BTMR_rCoolClbFlg_C
  Conversion1 : DataTypeConversion  OutDataTypeStr=uint8
  Data Type Conversion2 : DataTypeConversion  OutDataTypeStr=uint8
  Data Type Conversion5 : DataTypeConversion  OutDataTypeStr=uint8
  Relational Operator : RelationalOperator  Operator=>  OutDataTypeStr=boolean  RndMeth=Simplest
  Switch{1..4,8,11} (6 alike) : Switch  Criteria=u2 ~= 0
  BTMR_flgClntTempReq : Outport
  BTMR_tClntTempReq : Outport  Port=2
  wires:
  Constant5/1 -> Data Type Conversion2/1
  Data Type Conversion2/1 -> Switch2/1
  Relational Operator/1 -> Switch8/2, Switch1/2, Conversion1/1
  Switch3/1 -> Switch8/3
  Switch4/1 -> Switch2/3, Switch11/2
  Constant4/1 -> Switch3/1
  Constant10/1 -> Switch8/1
  Switch2/1 -> Switch1/3
  BTMR_flgBrsTempReq/1 -> Switch3/2, Switch2/2
  Switch11/1 -> Switch3/3
  Conversion1/1 -> Switch1/1
  Switch8/1 -> BTMR_tClntTempReq/1
  Switch1/1 -> BTMR_flgClntTempReq/1
  Constant7/1 -> Data Type Conversion5/1
  BTMR_flgClntTempReqMerge/1 -> Switch4/1
  Data Type Conversion5/1 -> Switch4/3
  Constant16/1 -> Switch11/3
  BTMR_tClntTempReqMerge/1 -> Switch11/1
  stCoolSts/1 -> Switch4/2
  Constant/1 -> Relational Operator/2
  Constant9/1 -> Relational Operator/1

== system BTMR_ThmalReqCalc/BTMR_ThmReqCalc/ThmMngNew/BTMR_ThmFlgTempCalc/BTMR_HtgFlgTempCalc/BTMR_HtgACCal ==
  Enable : EnablePort  StatesWhenEnabling=reset
  Constant1 : Constant  Value=BTMR_tHtgACTempReq_C
  Constant2 : Constant  Value=enmThmHeatFlg.ACTIVE  OutDataTypeStr=Enum: enmThmHeatFlg
  Data Type Conversion1 : DataTypeConversion  OutDataTypeStr=uint8
  BTMR_flgHtgTempReq : Outport  InitialOutput=0
  BTMR_tHtgTempReq : Outport  Port=2  InitialOutput=0
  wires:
  Constant1/1 -> BTMR_tHtgTempReq/1
  Data Type Conversion1/1 -> BTMR_flgHtgTempReq/1
  Constant2/1 -> Data Type Conversion1/1

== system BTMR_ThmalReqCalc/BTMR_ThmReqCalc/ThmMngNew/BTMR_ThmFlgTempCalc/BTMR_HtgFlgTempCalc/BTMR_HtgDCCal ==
  Enable : EnablePort  StatesWhenEnabling=reset
  Constant1 : Constant  Value=BTMR_tHtgDCTempReq_C
  Constant2 : Constant  Value=enmThmHeatFlg.ACTIVE  OutDataTypeStr=Enum: enmThmHeatFlg
  Data Type Conversion1 : DataTypeConversion  OutDataTypeStr=uint8
  BTMR_flgHtgTempReq : Outport  InitialOutput=0
  BTMR_tHtgTempReq : Outport  Port=2  InitialOutput=0
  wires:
  Data Type Conversion1/1 -> BTMR_flgHtgTempReq/1
  Constant1/1 -> BTMR_tHtgTempReq/1
  Constant2/1 -> Data Type Conversion1/1

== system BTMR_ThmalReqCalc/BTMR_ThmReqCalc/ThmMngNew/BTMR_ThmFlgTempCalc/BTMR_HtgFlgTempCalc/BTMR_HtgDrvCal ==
  Enable : EnablePort  StatesWhenEnabling=reset
  Constant2 : Constant  Value=enmThmHeatFlg.ACTIVE  OutDataTypeStr=Enum: enmThmHeatFlg
  Constant3 : Constant  Value=BTMR_tHtgDrvTempReq_C
  Data Type Conversion1 : DataTypeConversion  OutDataTypeStr=uint8
  BTMR_flgHtgTempReq : Outport  InitialOutput=0
  BTMR_tHtgTempReq : Outport  Port=2  InitialOutput=0
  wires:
  Constant2/1 -> Data Type Conversion1/1
  Data Type Conversion1/1 -> BTMR_flgHtgTempReq/1
  Constant3/1 -> BTMR_tHtgTempReq/1

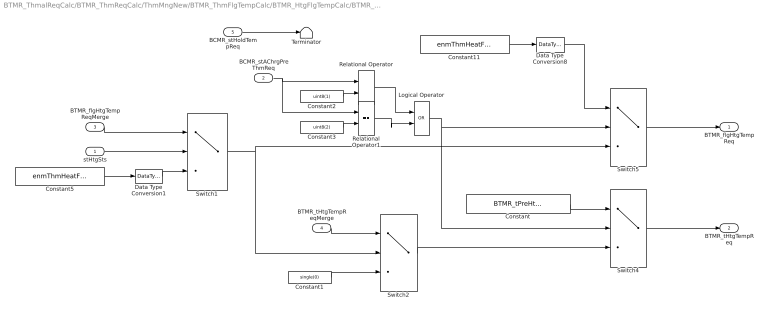
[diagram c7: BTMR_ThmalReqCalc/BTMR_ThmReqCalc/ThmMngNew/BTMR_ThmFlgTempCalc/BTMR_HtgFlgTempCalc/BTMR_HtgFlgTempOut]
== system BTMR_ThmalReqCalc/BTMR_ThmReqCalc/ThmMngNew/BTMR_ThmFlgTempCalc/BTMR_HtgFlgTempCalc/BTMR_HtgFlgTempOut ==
  stHtgSts : Inport
  BCMR_stAChrgPreThmReq : Inport  Port=2
  BTMR_flgHtgTempReqMerge : Inport  Port=3
  BTMR_tHtgTempReqMerge : Inport  Port=4
  BCMR_stHoldTempReq : Inport  Port=5
  Constant : Constant  Value=BTMR_tPreHtgTemp_C
  Constant1 : Constant  Value=single(0)
  Constant11 : Constant  Value=enmThmHeatFlg.INACTIVE  OutDataTypeStr=Enum: enmThmHeatFlg
  Constant2 : Constant  Value=uint8(1)
  Constant3 : Constant  Value=uint8(2)
  Constant5 : Constant  Value=enmThmHeatFlg.INACTIVE  OutDataTypeStr=Enum: enmThmHeatFlg
  Data Type Conversion1 : DataTypeConversion  OutDataTypeStr=uint8
  Data Type Conversion8 : DataTypeConversion  OutDataTypeStr=uint8
  Logical Operator : Logic  Operator=OR  AllPortsSameDT=off  OutDataTypeStr=boolean
  Relational Operator : RelationalOperator  Operator===  OutDataTypeStr=boolean  RndMeth=Simplest
  Relational Operator1 : RelationalOperator  Operator===  OutDataTypeStr=boolean  RndMeth=Simplest
  Switch{1..2,4..5} (4 alike) : Switch  Criteria=u2 ~= 0
  Terminator : Terminator
  BTMR_flgHtgTempReq : Outport
  BTMR_tHtgTempReq : Outport  Port=2
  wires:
  BTMR_flgHtgTempReqMerge/1 -> Switch1/1
  Constant1/1 -> Switch2/3
  Switch2/1 -> Switch4/3
  Logical Operator/1 -> Switch4/2, Switch5/2
  Data Type Conversion8/1 -> Switch5/1
  Switch4/1 -> BTMR_tHtgTempReq/1
  Switch5/1 -> BTMR_flgHtgTempReq/1
  Constant/1 -> Switch4/1
  Constant11/1 -> Data Type Conversion8/1
  Switch1/1 -> Switch5/3, Switch2/2
  BTMR_tHtgTempReqMerge/1 -> Switch2/1
  stHtgSts/1 -> Switch1/2
  Constant5/1 -> Data Type Conversion1/1
  Data Type Conversion1/1 -> Switch1/3
  BCMR_stHoldTempReq/1 -> Terminator/1
  Relational Operator/1 -> Logical Operator/1
  Constant2/1 -> Relational Operator/2
  BCMR_stAChrgPreThmReq/1 -> Relational Operator1/1, Relational Operator/1
  Constant3/1 -> Relational Operator1/2
  Relational Operator1/1 -> Logical Operator/2

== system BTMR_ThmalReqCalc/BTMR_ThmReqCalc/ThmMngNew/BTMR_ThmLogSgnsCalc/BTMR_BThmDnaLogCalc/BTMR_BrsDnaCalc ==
  BTMR_flgBrsLogSgns : Inport
  Bus Selector : BusSelector  OutputSignals=BTMR_flgBrsInTempSgns
  Bus Selector2 : BusSelector  OutputSignals=BTMR_flgBrsDnaTemp
  BTMR_flgBrsDna : Outport
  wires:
  Bus Selector2/1 -> BTMR_flgBrsDna/1  "<BTMR_flgBrsDnaTemp>"
  BTMR_flgBrsLogSgns/1 -> Bus Selector/1
  Bus Selector/1 -> Bus Selector2/1  "<BTMR_flgBrsInTempSgns>"

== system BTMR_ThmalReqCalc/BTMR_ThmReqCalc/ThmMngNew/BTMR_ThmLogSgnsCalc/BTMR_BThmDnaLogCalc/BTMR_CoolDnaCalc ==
  BTMR_flgCoolLogSgns : Inport
  Bus Selector : BusSelector  OutputSignals=BTMR_flgCoolNormTempSgns
  Bus Selector1 : BusSelector  OutputSignals=BTMR_flgCoolNormDnaTemp
  Bus Selector2 : BusSelector  OutputSignals=BTMR_flgCoolChrgTempSgns
  Bus Selector3 : BusSelector  OutputSignals=BTMR_flgCoolChrgDnaTemp
  BTMR_flgCoolNormDna : Outport
  BTMR_flgCoolChrgDna : Outport  Port=2
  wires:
  Bus Selector3/1 -> BTMR_flgCoolChrgDna/1  "<BTMR_flgCoolChrgDnaTemp>"
  Bus Selector2/1 -> Bus Selector3/1  "<BTMR_flgCoolChrgTempSgns>"
  Bus Selector/1 -> Bus Selector1/1  "<BTMR_flgCoolNormTempSgns>"
  BTMR_flgCoolLogSgns/1 -> Bus Selector/1, Bus Selector2/1
  Bus Selector1/1 -> BTMR_flgCoolNormDna/1  "<BTMR_flgCoolNormDnaTemp>"

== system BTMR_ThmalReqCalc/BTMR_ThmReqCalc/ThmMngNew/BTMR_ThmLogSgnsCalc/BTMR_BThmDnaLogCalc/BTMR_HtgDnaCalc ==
  BTMR_flgHtgLogSgns : Inport
  BTMR_flgSOCSgns : Inport  Port=2
  Bus Selector : BusSelector  OutputSignals=BTMR_flgHtgDCTempSgns
  Bus Selector1 : BusSelector  OutputSignals=BTMR_flgHtgDCDnaTemp
  Bus Selector2 : BusSelector  OutputSignals=BTMR_flgHtgACTempSgns
  Bus Selector3 : BusSelector  OutputSignals=BTMR_flgHtgACDnaTemp
  Bus Selector4 : BusSelector  OutputSignals=BTMR_flgHtgDrvTempSgns
  Bus Selector5 : BusSelector  OutputSignals=BTMR_flgHtgDrvDnaTemp
  Bus Selector6 : BusSelector  OutputSignals=BTMR_flgHtgDrvSOC
  Logical Operator1 : Logic  Operator=NOT  AllPortsSameDT=off  OutDataTypeStr=boolean
  Logical Operator3 : Logic  Operator=OR  AllPortsSameDT=off  OutDataTypeStr=boolean
  BTMR_flgHtgDCDna : Outport
  BTMR_flgHtgACDna : Outport  Port=2
  BTMR_flgHtgDrvDna : Outport  Port=3
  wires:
  Bus Selector1/1 -> BTMR_flgHtgDCDna/1  "<BTMR_flgHtgDCDnaTemp>"
  Bus Selector4/1 -> Bus Selector5/1  "<BTMR_flgHtgDrvTempSgns>"
  BTMR_flgHtgLogSgns/1 -> Bus Selector2/1, Bus Selector4/1, Bus Selector/1
  Bus Selector5/1 -> Logical Operator3/1  "<BTMR_flgHtgDrvDnaTemp>"
  Bus Selector/1 -> Bus Selector1/1  "<BTMR_flgHtgDCTempSgns>"
  Bus Selector2/1 -> Bus Selector3/1  "<BTMR_flgHtgACTempSgns>"
  Bus Selector3/1 -> BTMR_flgHtgACDna/1  "<BTMR_flgHtgACDnaTemp>"
  BTMR_flgSOCSgns/1 -> Bus Selector6/1
  Bus Selector6/1 -> Logical Operator1/1  "<BTMR_flgHtgDrvSOC>"
  Logical Operator3/1 -> BTMR_flgHtgDrvDna/1
  Logical Operator1/1 -> Logical Operator3/2

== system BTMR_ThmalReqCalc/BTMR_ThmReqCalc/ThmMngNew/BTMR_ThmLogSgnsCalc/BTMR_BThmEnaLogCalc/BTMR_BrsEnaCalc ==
  BTMR_flgBrsLogSgns : Inport
  Bus Selector : BusSelector  OutputSignals=BTMR_flgBrsEnaLogSgns
  Bus Selector1 : BusSelector  OutputSignals=BTMR_flgBrsEna
  BTMR_flgBrsEna : Outport
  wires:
  BTMR_flgBrsLogSgns/1 -> Bus Selector/1
  Bus Selector/1 -> Bus Selector1/1  "<BTMR_flgBrsEnaLogSgns>"
  Bus Selector1/1 -> BTMR_flgBrsEna/1  "<BTMR_flgBrsEna>"

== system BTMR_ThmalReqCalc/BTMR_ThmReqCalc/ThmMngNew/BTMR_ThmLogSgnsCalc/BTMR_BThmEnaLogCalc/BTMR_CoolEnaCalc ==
  BTMR_flgCoolLogSgns : Inport
  Bus Selector : BusSelector  OutputSignals=BTMR_flgCoolNormLogSgns
  Bus Selector1 : BusSelector  OutputSignals=BTMR_flgCoolNormEna
  Bus Selector2 : BusSelector  OutputSignals=BTMR_flgCoolChrgLogSgns
  Bus Selector3 : BusSelector  OutputSignals=BTMR_flgCoolChrgEna
  BTMR_flgCoolNormEna : Outport
  BTMR_flgCoolChrgEna : Outport  Port=2
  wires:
  Bus Selector1/1 -> BTMR_flgCoolNormEna/1  "<BTMR_flgCoolNormEna>"
  BTMR_flgCoolLogSgns/1 -> Bus Selector2/1, Bus Selector/1
  Bus Selector/1 -> Bus Selector1/1  "<BTMR_flgCoolNormLogSgns>"
  Bus Selector2/1 -> Bus Selector3/1  "<BTMR_flgCoolChrgLogSgns>"
  Bus Selector3/1 -> BTMR_flgCoolChrgEna/1  "<BTMR_flgCoolChrgEna>"

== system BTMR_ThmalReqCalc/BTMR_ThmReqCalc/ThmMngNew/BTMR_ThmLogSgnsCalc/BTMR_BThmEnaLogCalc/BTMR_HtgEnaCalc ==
  BTMR_flgHtgLogSgns : Inport
  BTMR_flgSOCSgns : Inport  Port=2
  Bus Selector : BusSelector  OutputSignals=BTMR_flgHtgDCLogSgns
  Bus Selector1 : BusSelector  OutputSignals=BTMR_flgHtgDCEna
  Bus Selector2 : BusSelector  OutputSignals=BTMR_flgHtgACLogSgns
  Bus Selector3 : BusSelector  OutputSignals=BTMR_flgHtgACEna
  Bus Selector4 : BusSelector  OutputSignals=BTMR_flgHtgDrvLogSgns
  Bus Selector5 : BusSelector  OutputSignals=BTMR_flgHtgDrvEna
  Bus Selector6 : BusSelector  OutputSignals=BTMR_flgHtgDrvSOC
  Logical Operator : Logic  AllPortsSameDT=off  OutDataTypeStr=boolean
  BTMR_flgHtgDCEna : Outport
  BTMR_flgHtgACEna : Outport  Port=2
  BTMR_flgHtgDrvEna : Outport  Port=3
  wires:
  Bus Selector3/1 -> BTMR_flgHtgACEna/1  "<BTMR_flgHtgACEna>"
  Bus Selector2/1 -> Bus Selector3/1  "<BTMR_flgHtgACLogSgns>"
  Bus Selector/1 -> Bus Selector1/1  "<BTMR_flgHtgDCLogSgns>"
  Bus Selector5/1 -> Logical Operator/1  "<BTMR_flgHtgDrvEna>"
  BTMR_flgHtgLogSgns/1 -> Bus Selector/1, Bus Selector4/1, Bus Selector2/1
  Bus Selector4/1 -> Bus Selector5/1  "<BTMR_flgHtgDrvLogSgns>"
  Bus Selector1/1 -> BTMR_flgHtgDCEna/1  "<BTMR_flgHtgDCEna>"
  BTMR_flgSOCSgns/1 -> Bus Selector6/1
  Logical Operator/1 -> BTMR_flgHtgDrvEna/1  "BTMR_flgHtgDrvSEna"
  Bus Selector6/1 -> Logical Operator/2  "<BTMR_flgHtgDrvSOC>"

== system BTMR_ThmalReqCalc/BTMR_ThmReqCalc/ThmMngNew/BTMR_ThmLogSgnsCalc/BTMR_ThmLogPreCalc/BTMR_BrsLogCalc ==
  BTMR_flgBMSStsSgns : Inport
  BTMR_flgSOCSgns : Inport  Port=2
  BTMR_flgBrsTempSgns : Inport  Port=3
  BTMR_BrsACLogCalc : Subsystem
  BTMR_BrsDCLogCalc : Subsystem
  BTMR_BrsDrvLogCalc : Subsystem
  BTMR_BrsEnaLogCalc : Subsystem
  Bus Creator1 : BusCreator  Inputs=4
  Bus Selector1 : BusSelector  OutputSignals=BTMR_flgBrsEnTempSgns,BTMR_flgBrsIntTempSgns
  BTMR_flgBrsLogSgns : Outport
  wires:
  Bus Selector1/2 -> BTMR_BrsDrvLogCalc/3(BTMR_flgBrsIntSgns), BTMR_BrsACLogCalc/3(BTMR_flgBrsIntSgns), BTMR_BrsDCLogCalc/3(BTMR_flgBrsIntSgns)  "<BTMR_flgBrsIntTempSgns>"
  Bus Selector1/1 -> BTMR_BrsDCLogCalc/2(BTMR_flgBrsEnSgns), BTMR_BrsDrvLogCalc/2(BTMR_flgBrsEnSgns), BTMR_BrsACLogCalc/2(BTMR_flgBrsEnSgns)  "<BTMR_flgBrsEnTempSgns>"
  BTMR_flgBMSStsSgns/1 -> BTMR_BrsDrvLogCalc/1(BTMR_flgBMSStsSgns), BTMR_BrsACLogCalc/1(BTMR_flgBMSStsSgns), BTMR_BrsDCLogCalc/1(BTMR_flgBMSStsSgns)
  BTMR_flgBrsTempSgns/1 -> BTMR_BrsEnaLogCalc/4(BTMR_flgBrsTempSgns), Bus Selector1/1
  BTMR_flgSOCSgns/1 -> BTMR_BrsDrvLogCalc/4(BTMR_flgSOCSgns)
  Bus Creator1/1 -> BTMR_flgBrsLogSgns/1  "BTMR_flgBrsLogSgns"
  BTMR_BrsDCLogCalc/1(BTMR_flgBrsDCLogSgns) -> BTMR_BrsEnaLogCalc/1(BTMR_flgBrsDCLogSgns), Bus Creator1/1
  BTMR_BrsACLogCalc/1(BTMR_flgBrsACLogSgns) -> BTMR_BrsEnaLogCalc/2(BTMR_flgBrsACLogSgns), Bus Creator1/2
  BTMR_BrsDrvLogCalc/1(BTMR_flgBrsDrvLogSgns) -> BTMR_BrsEnaLogCalc/3(BTMR_flgBrsDrvLogSgns), Bus Creator1/3
  BTMR_BrsEnaLogCalc/1(BTMR_flgBrsEnaLogSgns) -> Bus Creator1/4

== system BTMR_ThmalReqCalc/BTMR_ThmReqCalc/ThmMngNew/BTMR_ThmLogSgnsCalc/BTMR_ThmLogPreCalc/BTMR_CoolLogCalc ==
  BTMR_flgHtgLogSgns : Inport
  BTMR_flgThmEnaTempSgns : Inport  Port=2
  BTMR_CoolChrgLogCalc : Subsystem
  BTMR_CoolNormLogCalc : Subsystem
  Bus Creator : BusCreator  Inputs=2
  BTMR_flgCoolLogSgns : Outport
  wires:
  BTMR_flgHtgLogSgns/1 -> BTMR_CoolNormLogCalc/1(BTMR_flgHtgLogSgns), BTMR_CoolChrgLogCalc/1(BTMR_flgHtgLogSgns)
  BTMR_flgThmEnaTempSgns/1 -> BTMR_CoolNormLogCalc/2(BTMR_flgThmEnaTempSgns), BTMR_CoolChrgLogCalc/2(BTMR_flgThmEnaTempSgns)
  BTMR_CoolChrgLogCalc/1(BTMR_flgCoolChrgLogSgns) -> Bus Creator/2
  BTMR_CoolNormLogCalc/1(BTMR_flgCoolNormLogSgns) -> Bus Creator/1
  Bus Creator/1 -> BTMR_flgCoolLogSgns/1  "BTMR_flgCoolLogSgns"

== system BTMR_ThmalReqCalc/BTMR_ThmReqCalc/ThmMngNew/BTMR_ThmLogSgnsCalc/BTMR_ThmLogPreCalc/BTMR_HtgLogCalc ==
  BTMR_flgBrsLogSgns : Inport
  BTMR_flgThmEnaTempSgns : Inport  Port=2
  BTMR_HtgACLogCalc : Subsystem
  BTMR_HtgDCLogCalc : Subsystem
  BTMR_HtgDrvLogCalc : Subsystem
  Bus Creator : BusCreator  Inputs=3
  BTMR_flgHtgLogSgns : Outport
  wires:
  BTMR_HtgDCLogCalc/1(BTMR_flgHtgDCLogSgns) -> Bus Creator/1
  BTMR_flgThmEnaTempSgns/1 -> BTMR_HtgDrvLogCalc/2(BTMR_flgThmEnaTempSgns), BTMR_HtgACLogCalc/2(BTMR_flgThmEnaTempSgns), BTMR_HtgDCLogCalc/2(BTMR_flgThmEnaTempSgns)
  BTMR_HtgDrvLogCalc/1(BTMR_flgHtgDrvLogSgns) -> Bus Creator/3
  Bus Creator/1 -> BTMR_flgHtgLogSgns/1  "BTMR_flgHtgLogSgns"
  BTMR_HtgACLogCalc/1(BTMR_flgHtgACLogSgns) -> Bus Creator/2
  BTMR_flgBrsLogSgns/1 -> BTMR_HtgDrvLogCalc/1(BTMR_flgBrsLogSgns), BTMR_HtgACLogCalc/1(BTMR_flgBrsLogSgns), BTMR_HtgDCLogCalc/1(BTMR_flgBrsLogSgns)

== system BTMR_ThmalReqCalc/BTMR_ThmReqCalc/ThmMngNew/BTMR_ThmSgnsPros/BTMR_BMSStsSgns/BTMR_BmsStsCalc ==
  BMCR_stBmsModeCtrl : Inport
  COMR_bLeadAcidChgHvOn : Inport  Port=2
  Bus Creator : BusCreator  Inputs=4
  Data Type Conversion : DataTypeConversion  OutDataTypeStr=uint8
  Data Type Conversion1 : DataTypeConversion  OutDataTypeStr=uint8
  Data Type Conversion2 : DataTypeConversion  OutDataTypeStr=uint8
  Logical Operator1 : Logic  Operator=NOT  Inputs=3  AllPortsSameDT=off  OutDataTypeStr=boolean
  Logical Operator10 : Logic  Operator=OR  Inputs=3  AllPortsSameDT=off  OutDataTypeStr=boolean
  Logical Operator2 : Logic  AllPortsSameDT=off  OutDataTypeStr=boolean
  Logical Operator3 : Logic  Operator=NOT  AllPortsSameDT=off  OutDataTypeStr=boolean
  Relational Operator3 : RelationalOperator  Operator===  OutDataTypeStr=boolean  RndMeth=Simplest
  Relational Operator4 : RelationalOperator  Operator===  OutDataTypeStr=boolean  RndMeth=Simplest
  Relational Operator5 : RelationalOperator  Operator===  OutDataTypeStr=boolean  RndMeth=Simplest
  stBms_DChrg : Constant  Value=enmThmBmsSts.DCChrg  OutDataTypeStr=Enum: enmThmBmsSts
  stBms_DChrg1 : Constant  Value=enmThmBmsSts.ACChrg  OutDataTypeStr=Enum: enmThmBmsSts
  stBms_DChrg2 : Constant  Value=enmThmBmsSts.HvOn  OutDataTypeStr=Enum: enmThmBmsSts
  BTMR_flgBMSSgns : Outport
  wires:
  Data Type Conversion2/1 -> Relational Operator5/2
  BMCR_stBmsModeCtrl/1 -> Relational Operator3/1, Relational Operator5/1, Relational Operator4/1
  stBms_DChrg/1 -> Data Type Conversion/1
  Data Type Conversion1/1 -> Relational Operator4/2
  Logical Operator2/1 -> Bus Creator/3, Logical Operator10/3  "BTMR_flgBMSDrv"
  Relational Operator3/1 -> Bus Creator/1, Logical Operator10/1  "BTMR_flgBMSDChrg"
  Relational Operator4/1 -> Bus Creator/2, Logical Operator10/2  "BTMR_flgBMSAChrg"
  Logical Operator10/1 -> Logical Operator1/1
  Bus Creator/1 -> BTMR_flgBMSSgns/1
  Logical Operator1/1 -> Bus Creator/4  "BTMR_flgBMSOther"
  Relational Operator5/1 -> Logical Operator2/1  "BTMR_flgBMSHV"
  COMR_bLeadAcidChgHvOn/1 -> Logical Operator3/1
  Logical Operator3/1 -> Logical Operator2/2
  Data Type Conversion/1 -> Relational Operator3/2
  stBms_DChrg1/1 -> Data Type Conversion1/1
  stBms_DChrg2/1 -> Data Type Conversion2/1

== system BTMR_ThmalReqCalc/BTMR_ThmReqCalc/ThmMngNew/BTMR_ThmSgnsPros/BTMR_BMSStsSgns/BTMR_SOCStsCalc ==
  BSER_rSoc : Inport
  Bus Creator1 : BusCreator  Inputs=2
  Constant18 : Constant  Value=BTMR_r891HtgDrvSoc_C
  Constant21 : Constant  Value=BTMR_r891BrsDrvSoc_C
  Relational Operator6 : RelationalOperator  Operator=>  OutDataTypeStr=boolean  RndMeth=Simplest
  Relational Operator7 : RelationalOperator  Operator=>  OutDataTypeStr=boolean  RndMeth=Simplest
  BTMR_flgSOCSgns : Outport
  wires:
  Constant18/1 -> Relational Operator6/2
  BSER_rSoc/1 -> Relational Operator6/1, Relational Operator7/1
  Constant21/1 -> Relational Operator7/2
  Relational Operator7/1 -> Bus Creator1/1  "BTMR_flgBrsDrvSOC"
  Relational Operator6/1 -> Bus Creator1/2  "BTMR_flgHtgDrvSOC"
  Bus Creator1/1 -> BTMR_flgSOCSgns/1

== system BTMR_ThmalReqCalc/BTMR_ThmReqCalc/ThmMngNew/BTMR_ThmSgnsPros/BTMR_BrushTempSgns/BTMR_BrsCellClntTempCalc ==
  BSPR_tCellTempMax : Inport
  BSPR_tClntUsT : Inport  Port=2
  BSPR_tCellTempMin : Inport  Port=3
  BMSDebounceStartZero : AIWAYS_Powertrain_BMS_lib/Debounce & Delay/BMSDebounceStartZero
  Constant1 : Constant  Value=BTMR_tBrsCellClntDvtTemp_C
  Constant2 : Constant  Value=BTMR_tiTempBase_C
  Constant3 : Constant  Value=BTMR_tiTempDebs_C
  Constant4 : Constant  Value=BTMR_tBrsCellClntDvtTemp_C
  Logical Operator4 : Logic  AllPortsSameDT=off  OutDataTypeStr=boolean
  Relational Operator1 : RelationalOperator  Operator=<  OutDataTypeStr=boolean  RndMeth=Simplest
  Relational Operator2 : RelationalOperator  Operator=<  OutDataTypeStr=boolean  RndMeth=Simplest
  Subtract : Sum  Inputs=+-
  Subtract1 : Sum  Inputs=+-
  BTMR_flgBrsCellClntTemp : Outport
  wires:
  BMSDebounceStartZero/1 -> BTMR_flgBrsCellClntTemp/1
  Relational Operator2/1 -> Logical Operator4/2
  BSPR_tCellTempMin/1 -> Subtract/1
  Constant1/1 -> Relational Operator1/2
  Subtract/1 -> Relational Operator1/1
  Relational Operator1/1 -> Logical Operator4/1
  Logical Operator4/1 -> BMSDebounceStartZero/1
  Constant3/1 -> BMSDebounceStartZero/4, BMSDebounceStartZero/2
  Constant2/1 -> BMSDebounceStartZero/5, BMSDebounceStartZero/3
  BSPR_tCellTempMax/1 -> Subtract1/2
  BSPR_tClntUsT/1 -> Subtract1/1, Subtract/2
  Constant4/1 -> Relational Operator2/2
  Subtract1/1 -> Relational Operator2/1

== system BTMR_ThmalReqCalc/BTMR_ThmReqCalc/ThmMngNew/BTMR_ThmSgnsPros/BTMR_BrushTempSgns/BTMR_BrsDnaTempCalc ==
  BSPR_tCellTempMin : Inport
  BSPR_tCellTempMax : Inport  Port=2
  Add : Sum  Inputs=+-
  Add1 : Sum  Inputs=+-
  BMSDebounceStartZero : AIWAYS_Powertrain_BMS_lib/Debounce & Delay/BMSDebounceStartZero
  Constant1 : Constant  Value=BTMR_tiTempBase_C
  Constant2 : Constant  Value=BTMR_t891BrsDiffLv0Temp_C
  Constant3 : Constant  Value=BTMR_tiTempDebs_C
  Constant4 : Constant  Value=BTMR_tBrsMinCellTempThre_C
  Constant5 : Constant  Value=BTMR_tBrsMinCellTempDeb_C
  Logical Operator4 : Logic  Operator=OR  AllPortsSameDT=off  OutDataTypeStr=boolean
  Relational Operator1 : RelationalOperator  Operator=<=  OutDataTypeStr=boolean  RndMeth=Simplest
  Relational Operator2 : RelationalOperator  Operator=<=  OutDataTypeStr=boolean  RndMeth=Simplest
  BTMR_flgBrsDnaTemp : Outport
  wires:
  BSPR_tCellTempMin/1 -> Relational Operator1/1, Add/2
  BSPR_tCellTempMax/1 -> Add/1
  Logical Operator4/1 -> BMSDebounceStartZero/1
  Constant2/1 -> Relational Operator2/2
  Add/1 -> Relational Operator2/1
  BMSDebounceStartZero/1 -> BTMR_flgBrsDnaTemp/1
  Constant3/1 -> BMSDebounceStartZero/4, BMSDebounceStartZero/2
  Constant1/1 -> BMSDebounceStartZero/5, BMSDebounceStartZero/3
  Constant4/1 -> Add1/1
  Constant5/1 -> Add1/2
  Add1/1 -> Relational Operator1/2
  Relational Operator2/1 -> Logical Operator4/1
  Relational Operator1/1 -> Logical Operator4/2
